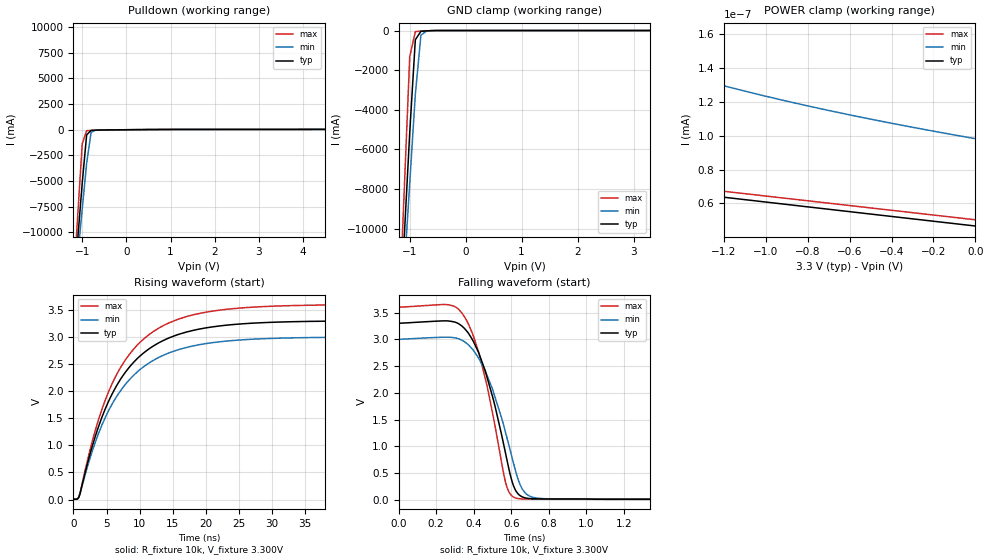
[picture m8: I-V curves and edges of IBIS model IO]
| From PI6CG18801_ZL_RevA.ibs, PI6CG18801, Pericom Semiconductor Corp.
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|   Model I/O
[Model]   IO
Model_type I/O_open_drain
Vinl = 990.00mV
Vinh = 2.3100V
Vref=3.300V
Vmeas=900mV
Rref=10k
| variable   typ   min   max
C_comp   0.680pF   0.679pF   0.681pF
[Voltage Range]   3.3000V   3.0000V   3.6000V
[POWER Clamp Reference]   3.3000V   3.0000V   3.6000V
[GND Clamp Reference]   0.0000V   0.0000V   0.0000V
[Pullup Reference]   3.3000V   3.0000V   3.6000V
[Pulldown Reference]   0.0000V   0.0000V   0.0000V
[Temperature Range]   25   85   -40
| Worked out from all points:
|   slope of the pulldown table from 0 to 0.495 V, typ, clamps not added: 29.4 ohm
|   GND clamp passes 1 mA (typ) near -0.51 V on its own axis
|   POWER clamp passes 1 mA (typ) near -2.41 V on its own axis
|   falling waveform, R_fixture 10k, V_fixture 3.300V: 20-80 % time 144ps typ, 155ps min, 132ps max; typ from 3.3 V to 0.008 V
|   rising waveform, R_fixture 10k, V_fixture 3.300V: 20-80 % time 7.86ns typ, 7.96ns min, 7.76ns max; typ from 0.008 V to 3.3 V
[GND Clamp]
| Voltage   I(typ)   I(min)   I(max)
-3.3V     -128.8A    -110.7A    -159.4A
-1.2V     -15.89A    -16.65A    -15.05A
-1.1V     -10.52A    -12.17A    -8.18A
-1V       -5.142A    -7.698A    -1.315A
-900mV    -465mA     -3.223A    -53.78mA
-800mV    -39.77mA   -236mA     -31.64mA
-700mV    -15.92mA   -25.22mA   -14.5mA
3.3V      46.73pA    104.9pA    46.2pA
[Power Clamp]
| Voltage   I(typ)   I(min)   I(max)
-3.3V     37.28A     21.05A     63A
-2.1V     2.093nA    205.7pA    518.6nA
-2V       118.8pA    161.6pA    3.936nA
-1.9V     74.64pA    155.6pA    105.7pA
-1.8V     72.28pA    151.3pA    75.81pA
-1.4V     66.55pA    136.1pA    70pA
-1V       60.86pA    123.2pA    64.4pA
-500mV    53.78pA    109.7pA    57.4pA
0V        46.73pA    98.19pA    50.4pA
[Pulldown]
| Voltage   I(typ)   I(min)   I(max)
-3.3V     -128.9A    -110.7A    -159.5A
-1.2V     -15.93A    -16.68A    -15.1A
-1.1V     -10.55A    -12.2A     -8.226A
-1V       -5.177A    -7.727A    -1.358A
-900mV    -498.1mA   -3.25A     -95.02mA
-700mV    -43.29mA   -47.79mA   -48.79mA
5.7V      39.52mA    39.58mA    50.4mA
5.9V      464.5mA    3.216A     62.08mA
6V        5.133A     7.683A     1.313A
6.1V      10.5A      12.15A     8.169A
6.2V      15.87A     16.62A     15.03A
6.6V      37.33A     34.49A     42.48A
[Falling Waveform]
R_fixture = 10k
V_fixture = 3.300V
V_fixture_min = 3.000V
V_fixture_max = 3.600V
|   Time   V(typ)   V(min)   V(max)
0s        3.3V       3V         3.6V
260ps     3.345V     3.04V      3.648V
350ps     3.206V     2.957V     3.426V
400ps     2.949V     2.787V     3.042V
460ps     2.424V     2.42V      2.293V
570ps     860.6mV    1.253V     319mV
615ps     234.9mV    641.3mV    43.93mV
660ps     50.83mV    192.9mV    14.66mV
740ps     15.73mV    28.31mV    11.89mV
2ns       8.331mV    9.427mV    7.012mV
[Rising Waveform]
R_fixture = 10k
V_fixture = 3.300V
V_fixture_min = 3.000V
V_fixture_max = 3.600V
|   Time   V(typ)   V(min)   V(max)
0s        7.615mV    8.561mV    6.464mV
800ps     38.19mV    40.35mV    35.39mV
2.8ns     962.9mV    875.2mV    1.054V
4ns       1.416V     1.283V     1.553V
5.8ns     1.937V     1.752V     2.126V
7.4ns     2.272V     2.056V     2.493V
11.5ns    2.788V     2.527V     3.052V
17ns      3.09V      2.805V     3.374V
33ns      3.282V     2.984V     3.58V
100ns     3.3V       3V         3.6V
[Ramp]
| variable   typ   min   max
dV/dt_r   1.97706V/7.8638n   1.79502V/7.9603n   2.15586V/7.7681n
dV/dt_f   1.97706V/144.09p   1.79502V/156.03p   2.15586V/131.83p
R_load = 10k
